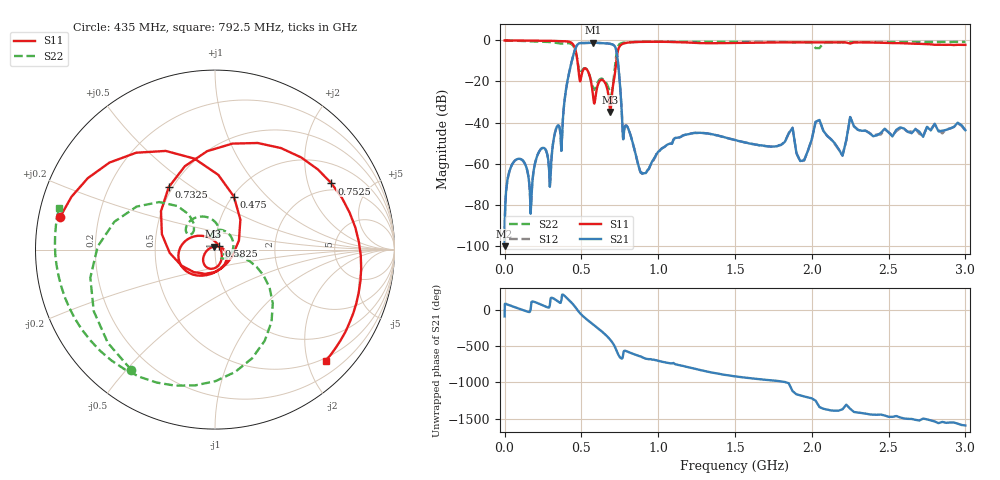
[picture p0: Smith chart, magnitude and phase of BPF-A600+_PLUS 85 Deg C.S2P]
! Mini-Circuits
! S2P DATA File Format
! Type: BAND PASS FILTER
! Model:BPF-A600+
! All S Parameters are in dB deg format
! TEST CONDITIONS: INPUT POWER = 0 dBm @ Temperature = + 85 deg C
! 401 Frequency points
# MHz S DB R 50
!FREQMAG(S11)PHS(S11)MAG(S21)PHS(S21)MAG(S12)PHS(S12)MAG(S22)PHS(S22)
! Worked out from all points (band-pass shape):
!   401 points, 500 kHz to 3 GHz, reference 50 ohm
!   highest |S21| = -1.07 dB at 575 MHz (marker M1); lowest = -100.3 dB at 500 kHz (marker M2)
!   |S21| within 3 dB of the highest: 460.6 MHz to 724.8 MHz (264.2 MHz wide, 44.6 % of centre)
!   lowest |S11| = -34.8 dB at 687.5 MHz (marker M3), VSWR 1.04, Z = 49.2 + j1.61 ohm
!   |S11| at or under -10 dB: 474.9 MHz to 727.9 MHz (253 MHz wide, 42.1 % of centre)
!   |S22| runs from -26.4 to 0.0 dB; largest |S21 - S12| = 0.0014
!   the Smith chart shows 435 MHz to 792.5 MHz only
!   S11 on the Smith chart (normalised r, x): 435 MHz: 0.06, +0.11; 475 MHz: 1.02, +0.67; 582.5 MHz: 1.04, +0.04; 732.5 MHz: 0.48, +0.41; 752.5 MHz: 1.71, +2.85; 792.5 MHz: 0.45, -2.34
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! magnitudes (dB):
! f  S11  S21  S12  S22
! 500 kHz  0.0  -100.3  -97.8  0.0
! 70 MHz  0.0  -58.4  -58.5  -0.1
! 170 MHz  -0.1  -84.5  -83.5  -0.4
! 235 MHz  -0.1  -53.1  -53.1  -0.6
! 295 MHz  -0.2  -71.3  -71.1  -0.8
! 435 MHz  -1.1  -10.9  -10.9  -1.8
! 475 MHz  -10.1  -2.0  -2.0  -9.9
! 502.5 MHz  -16.5  -1.2  -1.3  -15.0
! 575 MHz  -26.1  -1.1  -1.1  -22.9
! 582.5 MHz  -30.5  -1.1  -1.1  -24.1
! 637.5 MHz  -19.2  -1.3  -1.3  -18.7
! 687.5 MHz  -34.8  -1.6  -1.6  -25.6
! 732.5 MHz  -7.3  -7.0  -7.0  -4.8
! 752.5 MHz  -2.5  -22.6  -22.6  -1.6
! 772.5 MHz  -1.6  -48.1  -48.1  -1.1
! 792.5 MHz  -1.2  -41.5  -41.4  -0.9
! 890 MHz  -0.7  -64.7  -64.5  -0.7
! 1.01 GHz  -0.6  -53.7  -53.7  -0.6
! 1.51 GHz  -1.1  -48.7  -48.8  -0.7
! 2.025 GHz  -0.9  -39.7  -39.7  -3.7
! 2.525 GHz  -1.3  -46.8  -46.3  -0.8
! 3 GHz  -2.2  -43.8  -44.0  -0.7
